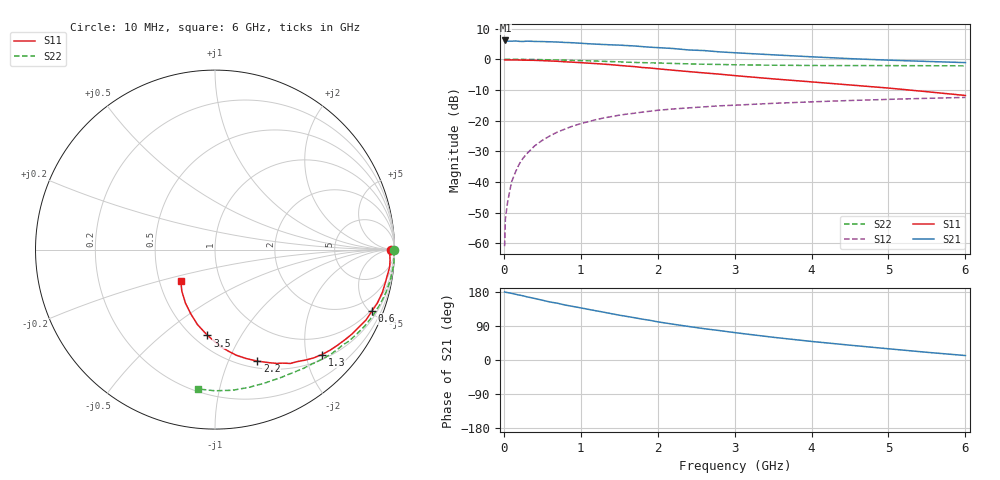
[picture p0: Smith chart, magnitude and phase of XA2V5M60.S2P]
! SIEMENS Discrete & RF Semiconductors
! BFY180
! Si NPN RF Bipolar Junction Transistor in MICRO-X
! VCE = 2.5 V  IC = 0.6 mA
! Common Emitter S-Parameters:  May  1997
# GHz  S  MA  R  50
!  f  S11  S21  S12  S22
! GHz  MAG  ANG  MAG  ANG  MAG  ANG  MAG  ANG
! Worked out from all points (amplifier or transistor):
!   36 points, 10 MHz to 6 GHz, reference 50 ohm
!   highest |S21| = 6.1 dB at 20 MHz (marker M1)
!   |S21| within 3 dB of that: start of sweep to 2.359 GHz
!   unconditionally stable (mu >= 1): 4.896 GHz to end of sweep
!   at 250 MHz: K = 0.06, MSG = 19.0 dB, |S12| = -32.2 dB
!   at 1.4 GHz: K = 0.42, MSG = 11.7 dB, |S12| = -18.7 dB
!   at 6 GHz: K = 1.04, MAG = 4.5 dB, |S12| = -12.4 dB
!   S11 on the Smith chart (normalised r, x): 10 MHz: 87, -14; 600 MHz: 0.89, -5.17; 1.3 GHz: 0.60, -2.31; 2.2 GHz: 0.58, -1.28; 3.5 GHz: 0.59, -0.73; 6 GHz: 0.64, -0.24
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0.01  0.9778 -0.2  1.962 179.8  0.0009 82.5  0.9991 -0.2
0.02  0.9799 -0.7  2.03 178.9  0.0025 89.2  0.9999 -0.5
0.05  0.9745 -1.8  1.978 177.9  0.0048 82.9  0.999 -1.2
0.1  0.9771 -3.5  1.976 175.9  0.01 88.7  0.9974 -2.4
0.2  0.9737 -7.3  1.963 171.3  0.0196 84.3  0.9974 -4.8
0.25  0.9694 -9.1  1.954 169.4  0.0245 83.3  0.9978 -6.0
0.4  0.9626 -14.3  1.958 162.4  0.0388 79.2  0.9927 -9.4
0.6  0.9394 -21.3  1.931 153.1  0.0566 74.0  0.9814 -14.1
0.8  0.9102 -28.4  1.882 144.9  0.0735 68.6  0.9675 -18.6
1.1  0.8663 -37.9  1.794 133.6  0.0965 60.9  0.944 -25.0
1.3  0.8343 -44.5  1.743 126.1  0.1109 56.5  0.9276 -29.0
1.5  0.7963 -50.6  1.704 118.3  0.1228 52.3  0.9098 -32.9
1.7  0.7606 -56.5  1.651 111.5  0.1323 48.5  0.8889 -36.6
2  0.7009 -64.1  1.551 100.7  0.1477 43.5  0.8715 -41.6
2.2  0.6647 -69.2  1.501 94.5  0.155 39.9  0.8569 -45.0
2.6  0.6011 -78.5  1.39 82.7  0.1678 34.6  0.8323 -50.7
3  0.5427 -86.5  1.28 72.3  0.1787 29.6  0.8152 -56.3
3.5  0.48 -95.0  1.184 60.0  0.1916 24.7  0.8016 -62.8
4  0.4288 -103.2  1.099 49.0  0.2026 19.7  0.7936 -69.4
4.5  0.3819 -110.8  1.026 39.1  0.2131 15.3  0.7905 -76.1
5.5  0.2966 -128.5  0.924 20.3  0.2313 6.7  0.7866 -90.0
6  0.2575 -138.0  0.884 11.8  0.2393 2.1  0.7821 -97.0
